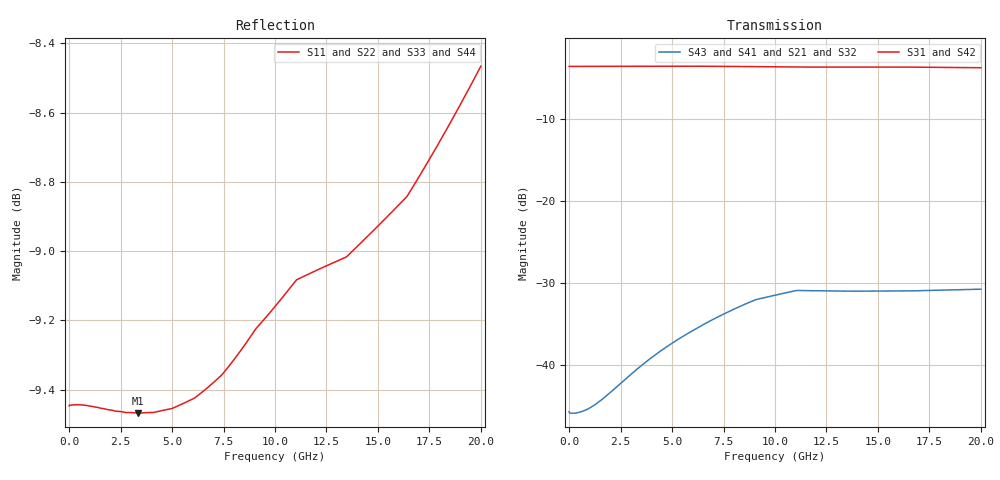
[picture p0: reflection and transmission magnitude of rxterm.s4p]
! Created Tue Jun 24 14:09:46 2014
# hz S db R 50
! 4 Port Network Data from SP1.SP block
! freq  dbS11  angS11  dbS12  angS12  dbS13  angS13  dbS14  angS14
!  dbS21  angS21  dbS22  angS22  dbS23  angS23  dbS24  angS24
!  dbS31  angS31  dbS32  angS32  dbS33  angS33  dbS34  angS34
!  dbS41  angS41  dbS42  angS42  dbS43  angS43  dbS44  angS44
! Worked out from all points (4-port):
!   2001 points, 1 MHz to 20 GHz, reference 50 ohm
!   strongest paths, dB at 1 MHz, 5.001 GHz, 10 GHz, 15 GHz, 20 GHz:
!     S31: -3.6, -3.5, -3.6, -3.7, -3.7
!     S42: -3.6, -3.5, -3.6, -3.7, -3.7
!     S43: -45.7, -37.3, -31.5, -31.0, -30.7
!     S41: -45.7, -37.3, -31.5, -31.0, -30.7
!     S21: -45.7, -37.3, -31.5, -31.0, -30.7
!     S32: -45.7, -37.3, -31.5, -31.0, -30.9
!   lowest |S11| = -9.5 dB at 3.361 GHz (marker M1), VSWR 2.01, Z = 24.9 - j0.967 ohm
!   |S11| at or under -10 dB: nowhere
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1000000  -9.45 -180.0  -45.67 -0.3  -3.57 -0.0  -45.67 -0.3
         -45.67 -0.3  -9.45 -180.0  -45.67 -0.3  -3.57 -0.0
         -3.57 -0.0  -45.67 -0.3  -9.45 -180.0  -45.67 -0.3
         -45.67 -0.3  -3.57 -0.0  -45.67 -0.3  -9.45 -180.0
1.180941e9  -9.45 -179.1  -44.93 23.9  -3.57 -0.5  -44.93 23.9
            -44.94 24.0  -9.45 -179.1  -44.94 24.0  -3.57 -0.5
            -3.57 -0.5  -44.93 23.9  -9.45 -179.1  -44.93 23.9
            -44.94 24.0  -3.57 -0.5  -44.94 24.0  -9.45 -179.1
3.360832e9  -9.47 -177.1  -40.35 45.4  -3.55 -1.5  -40.35 45.4
            -40.35 45.6  -9.47 -177.1  -40.35 45.6  -3.55 -1.5
            -3.55 -1.5  -40.35 45.4  -9.47 -177.1  -40.35 45.4
            -40.35 45.6  -3.55 -1.5  -40.35 45.6  -9.47 -177.1
6.710664e9  -9.39 -173.5  -34.82 42.7  -3.55 -3.3  -34.82 42.7
            -34.79 43.0  -9.39 -173.5  -34.79 43.0  -3.55 -3.3
            -3.55 -3.3  -34.82 42.7  -9.39 -173.5  -34.82 42.7
            -34.79 43.0  -3.55 -3.3  -34.79 43.0  -9.39 -173.5
9.890506e9  -9.17 -170.7  -31.57 25.1  -3.62 -4.9  -31.57 25.1
            -31.53 25.4  -9.17 -170.7  -31.53 25.4  -3.62 -4.9
            -3.62 -4.9  -31.57 25.1  -9.17 -170.7  -31.57 25.1
            -31.53 25.4  -3.62 -4.9  -31.53 25.4  -9.17 -170.7
1.110044e10  -9.08 -170.0  -30.94 16.0  -3.65 -5.3  -30.94 16.0
             -30.89 16.4  -9.08 -170.0  -30.89 16.4  -3.65 -5.3
             -3.65 -5.3  -30.94 16.0  -9.08 -170.0  -30.94 16.0
             -30.89 16.4  -3.65 -5.3  -30.89 16.4  -9.08 -170.0
2e10  -8.47 -162.4  -30.88 -16.7  -3.73 -10.1  -30.88 -16.7
      -30.73 -16.0  -8.46 -162.4  -30.73 -16.0  -3.74 -10.1
      -3.73 -10.1  -30.88 -16.7  -8.47 -162.4  -30.88 -16.7
      -30.73 -16.0  -3.74 -10.1  -30.73 -16.0  -8.46 -162.4
